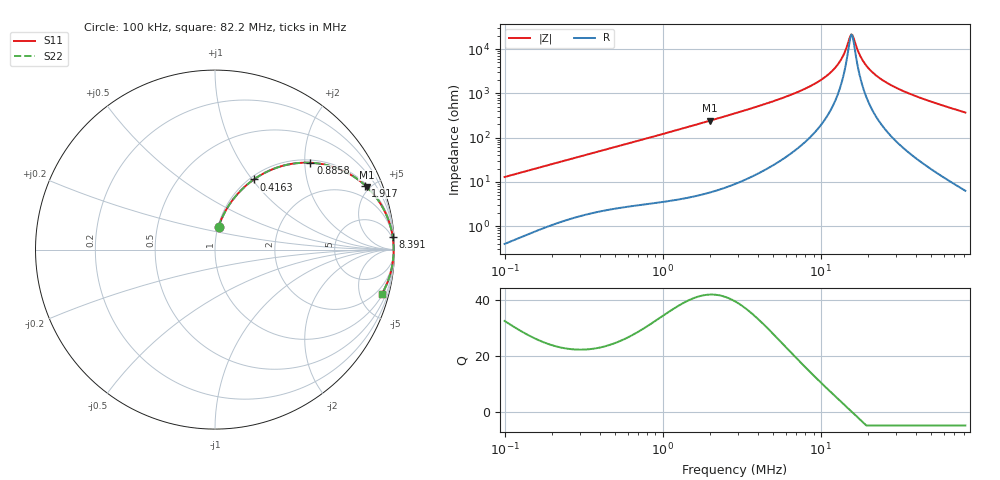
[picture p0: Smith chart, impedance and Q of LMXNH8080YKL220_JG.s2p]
! LMXNH8080YKL220_JG  S-PARAMETER MODEL  ( General Type )
! Model Generated by TAIYO YUDEN Corporation (http://www.ty-top.com)
! Version 1.0
! TAIYO YUDEN Control No. 191025NI43SB-FBB
! Copyright(c) 2019 TAIYO YUDEN CO.,LTD. All Rights Reserved.
! Product Description (link to TY-COMPAS)
! https://ds.yuden.co.jp/TYCOMPAS/or/detail?pn=LMXNH8080YKL220MJG&u=M
! Products Name : Inductors
! Characteristics :
!  Inductance : 22 uH , SRF(min) : 13 MHz , DC Resistance(max) : 0.0858 Ohm
!  Rated Current : Saturation :2400 mA , Temp Rise : 2200 mA
!  Case Size : 8.0 x 8.0 / 0.315 x 0.315 [mm/inch] , Thickness : 4 / 0.157 [mm/inch]
!  (Conditions: Temperature = 25 degC , DC Bias Current/Voltage = 0A / 0V)
! External Node Assignments :
!  1  o---GGG---o  2
! GND o---------o GND
! Frequency Range : 0.1MHz  -  82.198079MHz  [ 402 STEP ]
# MHz S RI R 50
! Freq[MHz].  S11 Real  S11 Imag  S21 Real  S21 Imag  S12 Real  S12 Imag  S22 Real  S22 Imag
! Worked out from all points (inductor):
!   401 points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, 100 kHz to 82.2 MHz, reference 50 ohm
!   read as one part in series: L = 20.3 uH near 103.4 kHz
!   highest Q = 42.1 at 1.982 MHz (marker M1), where L = 19.3 uH
!   self-resonance near 15.61 MHz
!   S11 on the Smith chart (normalised r, x): 100 kHz: 1.01, +0.26; 416.3 kHz: 1.04, +1.02; 885.8 kHz: 1.07, +2.13; 1.917 MHz: 1.11, +4.64; 8.391 MHz: 3, +28; 82.2 MHz: 1.13, -7.38
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0.1  0.0199 0.1253  0.9801 -0.1253  0.9801 -0.1253  0.0199 0.1253
0.307779  0.1382 0.3234  0.8618 -0.3234  0.8618 -0.3234  0.1382 0.3234
0.416302  0.2167 0.3911  0.7833 -0.3911  0.7833 -0.3911  0.2167 0.3911
0.885789  0.5318 0.4838  0.4682 -0.4838  0.4682 -0.4838  0.5318 0.4838
0.947281  0.5638 0.4812  0.4362 -0.4812  0.4362 -0.4812  0.5638 0.4812
1.916634  0.8378 0.357  0.1622 -0.357  0.1622 -0.357  0.8378 0.357
1.982045  0.8466 0.3487  0.1534 -0.3487  0.1534 -0.3487  0.8466 0.3487
2.867021  0.9204 0.2584  0.0796 -0.2584  0.0796 -0.2584  0.9204 0.2584
5.424287  0.9768 0.1323  0.0232 -0.1323  0.0232 -0.1323  0.9768 0.1323
8.390903  0.9902 0.0703  0.00981 -0.0703  0.00981 -0.0703  0.9902 0.0703
8.824095  0.9911 0.0641  0.00894 -0.0641  0.00894 -0.0641  0.9911 0.0641
10.79235  0.9937 0.0404  0.00635 -0.0404  0.00635 -0.0404  0.9937 0.0404
12.55164  0.9948 0.0237  0.00522 -0.0237  0.00522 -0.0237  0.9948 0.0237
13.65011  0.9951 0.0147  0.00485 -0.0147  0.00485 -0.0147  0.9951 0.0147
15.6111  0.9954 0.000403  0.00461 -0.000403  0.00461 -0.000403  0.9954 0.000403
16.14387  0.9954 -0.00316  0.00461 0.00316  0.00461 0.00316  0.9954 -0.00316
17.55672  0.9953 -0.0121  0.00474 0.0121  0.00474 0.0121  0.9953 -0.0121
19.4163  0.9949 -0.0229  0.00511 0.0229  0.00511 0.0229  0.9949 -0.0229
22.20566  0.994 -0.0377  0.006 0.0377  0.006 0.0377  0.994 -0.0377
27.15873  0.9917 -0.0611  0.00832 0.0611  0.00832 0.0611  0.9917 -0.0611
42.72309  0.9799 -0.1233  0.0201 0.1233  0.0201 0.1233  0.9799 -0.1233
82.19808  0.928 -0.2501  0.072 0.2501  0.072 0.2501  0.928 -0.2501
